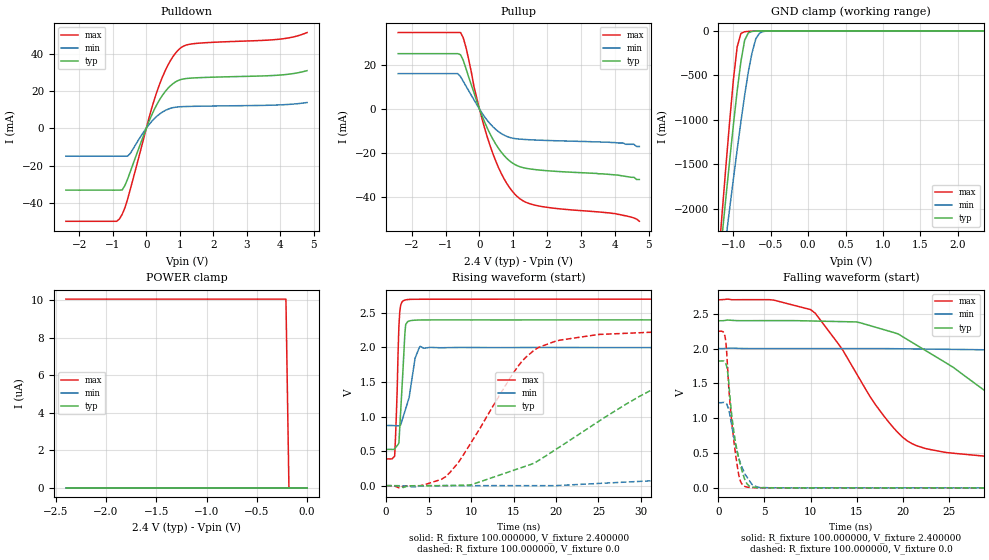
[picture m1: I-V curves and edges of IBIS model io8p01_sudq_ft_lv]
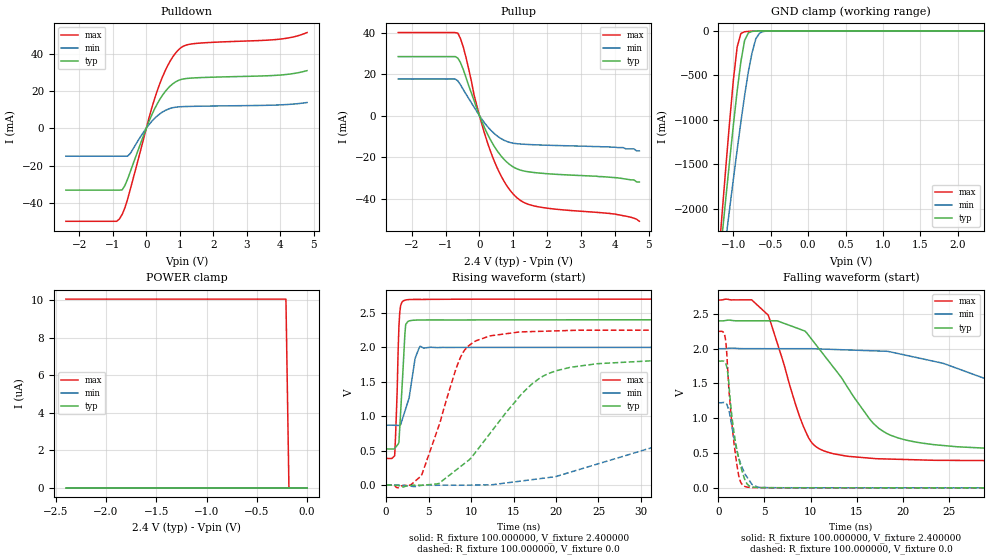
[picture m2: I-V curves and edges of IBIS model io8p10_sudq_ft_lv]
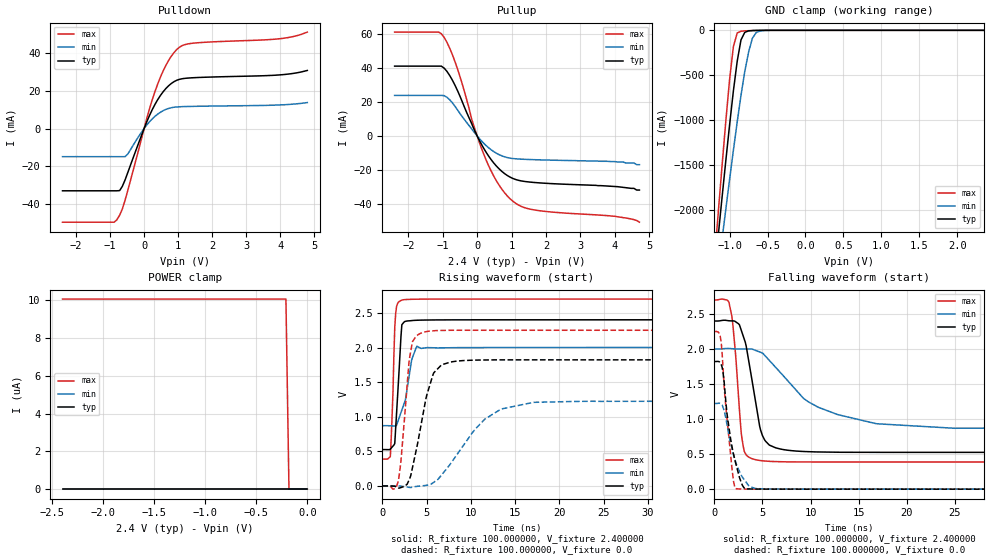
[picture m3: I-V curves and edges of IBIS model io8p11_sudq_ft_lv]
|   stm32f0_440_ufqfpn32 IBIS Model
[IBIS ver]   4.2
[File name]  stm32f0_440_ufqfpn32.ibs
[File Rev]   1.0
[Date]   15-5-2013
[Source] Data Created at STMicroelectronics
[Notes]   File originated from ELDO simulations.
[Disclaimer]  This information is for modeling purpose only and is
   not guaranted. The information is subject to change without
   notice.
[Copyright] Copyright 2015 STMicroelectronics Inc.
[Component] stm32f0_440_ufqfpn32
[Manufacturer] STMicroelectronics
[Package]
| variable   typ   min   max
R_pkg   0.0   NA   NA
L_pkg   0.0H   NA   NA
C_pkg   0.0F   NA   NA
[Pin] signal_name  model_name   R_pin   L_pin   C_pin
0   VSS_VSSA   GND   NA   NA   NA
1   VDD   POWER   0.03449   2.11E-09   6E-14
2   PF0   io8p_sudq_ft   0.029020556   1.54333E-09   3.22222E-14
3   PF1   io8p_sudq_ft   0.025738889   1.20333E-09   1.55556E-14
4   NRST  ioreset_tc_v33   0.024645   1.09E-09   1E-14
5   VDDA  POWER   0.024645   1.09E-09   1E-14
6   PA0   io8p_sudq_ft   0.025738889   1.20333E-09   1.55556E-14
7   PA1   io8p_sudq_ft   0.029020556   1.54333E-09   3.22222E-14
8   PA2   io8p_sudq_ft   0.03449   2.11E-09   6E-14
9   PA3   io8p_sudq_ft   0.03449   2.11E-09   6E-14
10   PA4   io8p_sudq_ft   0.029020556   1.54333E-09   3.22222E-14
11   PA5   io8p_sudq_ft   0.025738889   1.20333E-09   1.55556E-14
12   PA6   io8p_sudq_ft   0.024645   1.09E-09   1E-14
13   PA7   io8p_sudq_ft   0.024645   1.09E-09   1E-14
14   PB0   io8p_sudq_ft   0.025738889   1.20333E-09   1.55556E-14
15   PB1   io8p_sudq_ft   0.029020556   1.54333E-09   3.22222E-14
16   PB2   io8p_sudq_ft   0.03449   2.11E-09   6E-14
17   VDD   POWER   0.03449   2.11E-09   6E-14
18   PA8   io8p_sudq_ft   0.029020556   1.54333E-09   3.22222E-14
19   PA9   io8p_sudq_ft   0.025738889   1.20333E-09   1.55556E-14
20   PA10  io8p_sudq_ft   0.024645   1.09E-09   1E-14
21   PA11  io8p_sudq_ft   0.024645   1.09E-09   1E-14
22   PA12  io8p_sudq_ft   0.025738889   1.20333E-09   1.55556E-14
23   PA13  io8p_sudq_ft   0.029020556   1.54333E-09   3.22222E-14
24   PA14  io8p_sudq_ft   0.03449   2.11E-09   6E-14
25   PA15  io8p_sudq_ft   0.03449   2.11E-09   6E-14
26   PB3   io8p_sudq_ft   0.029020556   1.54333E-09   3.22222E-14
27   PB4   io8p_sudq_ft   0.025738889   1.20333E-09   1.55556E-14
28   PB5   io8p_sudq_ft   0.024645   1.09E-09   1E-14
29   PB6   io8p_sudq_i2cin_lv_ft   0.024645   1.09E-09   1E-14
30   PB7   io8p_sudq_i2cin_lv_ft   0.025738889   1.20333E-09   1.55556E-14
31   BOOT0 vpp_test_hv   0.029020556   1.54333E-09   3.22222E-14
32   PB8   io8p_sudq_i2cin_lv_ft   0.03449   2.11E-09   6E-14
[Model Selector] io8p_sudq_ft
io8p01_sudq_ft_pd_lv  "SPEED01 2P0V, PD=40kOhm"
io8p01_sudq_ft_pu_lv  "SPEED01 2P0V, PU=40kOhm"
io8p01_sudq_ft_lv  "SPEED01 2P0V"
io8p10_sudq_ft_pd_lv  "SPEED10 2P0V, PD=40kOhm"
io8p10_sudq_ft_pu_lv  "SPEED10 2P0V, PU=40kOhm"
io8p10_sudq_ft_lv  "SPEED10 2P0V"
io8p11_sudq_ft_pd_lv  "SPEED11 2P0V, PD=40kOhm"
io8p11_sudq_ft_pu_lv  "SPEED11 2P0V, PU=40kOhm"
io8p11_sudq_ft_lv  "SPEED11 2P0V"
io8p01_sudq_ft_pd  "SPEED01, PD=40kOhm"
io8p01_sudq_ft_pu  "SPEED01, PU=40kOhm"
io8p01_sudq_ft  "SPEED01"
io8p10_sudq_ft_pd  "SPEED10, PD=40kOhm"
io8p10_sudq_ft_pu  "SPEED10, PU=40kOhm"
io8p10_sudq_ft  "SPEED10"
io8p11_sudq_ft_pd  "SPEED11, PD=40kOhm"
io8p11_sudq_ft_pu  "SPEED11, PU=40kOhm"
io8p11_sudq_ft  "SPEED11"
[Model Selector] io8p_sudq_i2cin_lv_ft
io8p01_sudq_i2cin_lv_ft_pd_lv  "SPEED01 2P0V, PD=40kOhm"
io8p01_sudq_i2cin_lv_ft_pu_lv  "SPEED01 2P0V, PU=40kOhm"
io8p01_sudq_i2cin_lv_ft_lv  "SPEED01 2P0V"
io8p10_sudq_i2cin_lv_ft_pd_lv  "SPEED10 2P0V, PD=40kOhm"
io8p10_sudq_i2cin_lv_ft_pu_lv  "SPEED10 2P0V, PU=40kOhm"
io8p10_sudq_i2cin_lv_ft_lv  "SPEED10 2P0V"
io8p11_sudq_i2cin_lv_ft_pd_lv  "SPEED11 2P0V, PD=40kOhm"
io8p11_sudq_i2cin_lv_ft_pu_lv  "SPEED11 2P0V, PU=40kOhm"
io8p11_sudq_i2cin_lv_ft_lv  "SPEED11 2P0V"
io8p01_sudq_i2cin_lv_ft_pd  "SPEED01, PD=40kOhm"
io8p01_sudq_i2cin_lv_ft_pu  "SPEED01, PU=40kOhm"
io8p01_sudq_i2cin_lv_ft  "SPEED01"
io8p10_sudq_i2cin_lv_ft_pd  "SPEED10, PD=40kOhm"
io8p10_sudq_i2cin_lv_ft_pu  "SPEED10, PU=40kOhm"
io8p10_sudq_i2cin_lv_ft  "SPEED10"
io8p11_sudq_i2cin_lv_ft_pd  "SPEED11, PD=40kOhm"
io8p11_sudq_i2cin_lv_ft_pu  "SPEED11, PU=40kOhm"
io8p11_sudq_i2cin_lv_ft  "SPEED11"
[Model Selector] ioreset_tc_v33
ioreset_tc_v33_pu_lv  "IORESET 2V + PU=40kOhm"
ioreset_tc_v33_nopu_lv  "IORESET 2V"
ioreset_tc_v33_pu  "IORESET + PU=40kOhm"
ioreset_tc_v33_nopu  "IORESET"
[Model Selector] vpp_test_hv
vpp_test_hv_3p3  "Input Buffer"
vpp_test_hv_2p4  "Input Buffer 2P0V"
| Models and submodels in the file (42): io8p01_sudq_ft_pd_lv (I/O), io8p01_sudq_ft_pu_lv (I/O), io8p01_sudq_ft_lv (I/O), io8p10_sudq_ft_pd_lv (I/O), io8p10_sudq_ft_pu_lv (I/O), io8p10_sudq_ft_lv (I/O), io8p11_sudq_ft_pd_lv (I/O), io8p11_sudq_ft_pu_lv (I/O), io8p11_sudq_ft_lv (I/O), io8p01_sudq_ft_pd (I/O), io8p01_sudq_ft_pu (I/O), io8p01_sudq_ft (I/O), io8p10_sudq_ft_pd (I/O), io8p10_sudq_ft_pu (I/O), io8p10_sudq_ft (I/O), io8p11_sudq_ft_pd (I/O), io8p11_sudq_ft_pu (I/O), io8p11_sudq_ft (I/O), io8p01_sudq_i2cin_lv_ft_pd_lv (I/O), io8p01_sudq_i2cin_lv_ft_pu_lv (I/O), io8p01_sudq_i2cin_lv_ft_lv (I/O), io8p10_sudq_i2cin_lv_ft_pd_lv (I/O), io8p10_sudq_i2cin_lv_ft_pu_lv (I/O), io8p10_sudq_i2cin_lv_ft_lv (I/O), io8p11_sudq_i2cin_lv_ft_pd_lv (I/O), io8p11_sudq_i2cin_lv_ft_pu_lv (I/O), io8p11_sudq_i2cin_lv_ft_lv (I/O), io8p01_sudq_i2cin_lv_ft_pd (I/O), io8p01_sudq_i2cin_lv_ft_pu (I/O), io8p01_sudq_i2cin_lv_ft (I/O), io8p10_sudq_i2cin_lv_ft_pd (I/O), io8p10_sudq_i2cin_lv_ft_pu (I/O), io8p10_sudq_i2cin_lv_ft (I/O), io8p11_sudq_i2cin_lv_ft_pd (I/O), io8p11_sudq_i2cin_lv_ft_pu (I/O), io8p11_sudq_i2cin_lv_ft (I/O), ioreset_tc_v33_pu_lv (I/O_open_drain), ioreset_tc_v33_nopu_lv (I/O_open_drain), ioreset_tc_v33_pu (I/O_open_drain), ioreset_tc_v33_nopu (I/O_open_drain), vpp_test_hv_2p4 (Input), vpp_test_hv_3p3 (Input)
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|   Model io8p01_sudq_ft_lv
[Model]  io8p01_sudq_ft_lv
Model_type I/O
Polarity   Non-Inverting
Enable   Active-Low
Vinl =   0.720000V
Vinh =   1.680000V
Vmeas =  1.200000V
Cref =   50.000000pF
Rref =   100.000000M
Vref =   0.0V
C_comp   1.970100pF   1.887900pF   2.069400pF
[Temperature Range]   25.000000   0.125000k   -40.000000
[Pullup Reference]   2.400000V   2.000000V   2.700000V
[Pulldown Reference]   0.0V   0.0V   0.0V
[POWER Clamp Reference]   2.400000V   2.000000V   2.700000V
[GND Clamp Reference]   0.0V   0.0V   0.0V
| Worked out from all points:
|   slope of the pulldown table from 0 to 0.36 V, typ, clamps not added: 25.5 ohm
|   slope of the pullup table from 0 to 0.36 V, typ, clamps not added: 28.4 ohm
|   GND clamp passes 1 mA (typ) near -0.64 V on its own axis
|   rising waveform, R_fixture 100.000000, V_fixture 2.400000: 20-80 % time 499ps typ, 1.06ns min, 336ps max; typ from 0.525 V to 2.4 V
|   rising waveform, R_fixture 100.000000, V_fixture 0.0: 20-80 % time 14.5ns typ, 43.7ns min, 6.87ns max; typ from 0 V to 1.82 V
|   falling waveform, R_fixture 100.000000, V_fixture 2.400000: 20-80 % time 13ns typ, 32.3ns min, 7.05ns max; typ from 2.4 V to 0.525 V
|   falling waveform, R_fixture 100.000000, V_fixture 0.0: 20-80 % time 1.16ns typ, 1.39ns min, 931ps max; typ from 1.82 V to 0 V
[Pulldown]
|Voltage   I(typ)   I(min)   I(max)
-2.4V     -33.16mA   -14.98mA   -49.86mA
-880mV    -33.16mA   -14.98mA   -49.86mA
-800mV    -33.16mA   -14.98mA   -48.55mA
-640mV    -30.75mA   -14.98mA   -42.76mA
-480mV    -23.43mA   -13.57mA   -32.92mA
80mV      3.651mA    1.905mA    5.506mA
400mV     15.37mA    7.665mA    23.73mA
720mV     22.75mA    10.69mA    36.23mA
1.04V     26.18mA    11.57mA    43.27mA
1.52V     27.09mA    11.81mA    45.55mA
4V        28.55mA    12.55mA    47.81mA
4.8V      30.9mA     13.81mA    51.31mA
[Pullup]
|Voltage   I(typ)   I(min)   I(max)
-2.4V     25.21mA    16.13mA    34.79mA
-640mV    25.21mA    16.13mA    34.79mA
-560mV    24.72mA    14.75mA    34.79mA
-400mV    18.51mA    10.48mA    28.09mA
-160mV    7.322mA    4.15mA     10.02mA
80mV      -3.229mA   -1.94mA    -4.736mA
400mV     -13.82mA   -8.081mA   -20.45mA
800mV     -22.31mA   -12.38mA   -33.66mA
1.2V      -26.24mA   -13.65mA   -40.83mA
1.76V     -27.69mA   -14.12mA   -44.07mA
4V        -29.9mA    -15.2mA    -47.5mA
4.72V     -32mA      -17mA      -51mA
[GND_clamp]
|Voltage   I(typ)   I(min)   I(max)
-2.4V     -9.788A    -9.782A    -9.734A
-1.2V     -2.718A    -3.02A     -2.568A
-1.15V    -2.29A     -2.675A    -2.036A
-1.1V     -1.868A    -2.333A    -1.515A
-1.05V    -1.454A    -1.995A    -1.012A
-950mV    -674.5mA   -1.337A    -180.5mA
-900mV    -345.2mA   -1.023A    -29.72mA
-850mV    -106.4mA   -726mA     -10.13mA
-750mV    -6.396mA   -244mA     -4.026mA
-700mV    -2.558mA   -88.61mA   -2.329mA
-600mV    -416uA     -7.739mA   -368uA
2.35V     0A         0A         0A
[POWER_clamp]
|Voltage   I(typ)   I(min)   I(max)
-2.4V     0A         0A         10.06uA
-210mV    0A         0A         10.06uA
-180mV    0A         0A         0A
0V        0A         0A         0A
[Ramp]
| variable   typ   min   max
dV/dt_r  1.09308/14.53591n   0.73368/43.60005n   1.34946/6.86189n
dV/dt_f  1.12469/12.94342n   0.67781/32.23620n   1.38756/7.04174n
R_load = 100.000000
[Rising Waveform]
R_fixture= 100.000000
V_fixture= 2.400000
V_fixture_min= 2.000000
V_fixture_max= 2.700000
|time   V(typ)   V(min)   V(max)
0s        525.2mV    870.3mV    387.4mV
1.001ns   533.4mV    868.6mV    427.9mV
1.301ns   580.2mV    867mV      1.396V
1.502ns   618.9mV    866.4mV    2.308V
1.702ns   1.058V     877.1mV    2.607V
2.202ns   2.2V       1.075V     2.686V
2.703ns   2.383V     1.274V     2.696V
3.403ns   2.395V     1.844V     2.698V
4.004ns   2.398V     2.016V     2.698V
49.85ns   2.4V       2V         2.7V
[Rising Waveform]
R_fixture= 100.000000
V_fixture= 0.0
V_fixture_min= 0.0
V_fixture_max= 0.0
|time   V(typ)   V(min)   V(max)
0s        1.81nV     16.19nV    1.388nV
7.007ns   1.867mV    817.4uV    130.2mV
16.52ns   286.2mV    456uV      1.866V
20.02ns   528mV      1.164mV    2.095V
25.03ns   931.2mV    32.13mV    2.189V
37.04ns   1.629V     132.6mV    2.24V
54.55ns   1.791V     444.2mV    2.251V
84.08ns   1.821V     947.3mV    2.249V
106.1ns   1.822V     1.128V     2.249V
249.2ns   1.822V     1.223V     2.249V
[Falling Waveform]
R_fixture= 100.000000
V_fixture= 2.400000
V_fixture_min= 2.000000
V_fixture_max= 2.700000
|time   V(typ)   V(min)   V(max)
0s        2.4V       2V         2.7V
10.01ns   2.397V     2V         2.56V
15.02ns   2.383V     2V         1.637V
20.02ns   2.171V     1.997V     726.6mV
29.03ns   1.387V     1.983V     453.9mV
37.04ns   789.8mV    1.94V      415.8mV
52.55ns   592.4mV    1.669V     394.5mV
72.57ns   546.2mV    1.209V     388.6mV
99.1ns    528mV      969.1mV    387.4mV
249.2ns   525.2mV    870.3mV    387.4mV
[Falling Waveform]
R_fixture= 100.000000
V_fixture= 0.0
V_fixture_min= 0.0
V_fixture_max= 0.0
|time   V(typ)   V(min)   V(max)
0s        1.822V     1.223V     2.249V
700.7ps   1.802V     1.223V     2.18V
800.8ps   1.785V     1.216V     2.097V
1.001ns   1.655V     1.166V     1.704V
1.201ns   1.378V     1.071V     1.289V
1.902ns   616.6mV    591.6mV    436.6mV
2.302ns   369.3mV    388.2mV    131.7mV
2.903ns   108.1mV    191.2mV    18.1mV
4.705ns   2.197mV    4.103mV    1.139mV
49.85ns   1.81nV     16.19nV    1.388nV
|   Model io8p10_sudq_ft_lv
[Model]  io8p10_sudq_ft_lv
Model_type I/O
Polarity   Non-Inverting
Enable   Active-Low
Vinl =   0.720000V
Vinh =   1.680000V
Vmeas =  1.200000V
Cref =   50.000000pF
Rref =   100.000000M
Vref =   0.0V
C_comp   1.970100pF   1.887900pF   2.069400pF
[Temperature Range]   25.000000   0.125000k   -40.000000
[Pullup Reference]   2.400000V   2.000000V   2.700000V
[Pulldown Reference]   0.0V   0.0V   0.0V
[POWER Clamp Reference]   2.400000V   2.000000V   2.700000V
[GND Clamp Reference]   0.0V   0.0V   0.0V
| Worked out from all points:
|   slope of the pulldown table from 0 to 0.36 V, typ, clamps not added: 25.5 ohm
|   slope of the pullup table from 0 to 0.36 V, typ, clamps not added: 28.4 ohm
|   GND clamp passes 1 mA (typ) near -0.64 V on its own axis
|   rising waveform, R_fixture 100.000000, V_fixture 2.400000: 20-80 % time 501ps typ, 1.06ns min, 336ps max; typ from 0.525 V to 2.4 V
|   rising waveform, R_fixture 100.000000, V_fixture 0.0: 20-80 % time 7.32ns typ, 21.7ns min, 3.52ns max; typ from 0 V to 1.82 V
|   falling waveform, R_fixture 100.000000, V_fixture 2.400000: 20-80 % time 6.27ns typ, 18.5ns min, 3.33ns max; typ from 2.4 V to 0.525 V
|   falling waveform, R_fixture 100.000000, V_fixture 0.0: 20-80 % time 1.16ns typ, 1.4ns min, 914ps max; typ from 1.82 V to 0 V
[Pulldown]
|Voltage   I(typ)   I(min)   I(max)
-2.4V     -33.16mA   -14.98mA   -49.86mA
-880mV    -33.16mA   -14.98mA   -49.86mA
-800mV    -33.16mA   -14.98mA   -48.55mA
-640mV    -30.75mA   -14.98mA   -42.76mA
-480mV    -23.43mA   -13.57mA   -32.92mA
80mV      3.651mA    1.905mA    5.506mA
400mV     15.37mA    7.665mA    23.73mA
720mV     22.75mA    10.69mA    36.23mA
1.04V     26.18mA    11.57mA    43.27mA
1.52V     27.09mA    11.81mA    45.55mA
4V        28.55mA    12.55mA    47.81mA
4.8V      30.9mA     13.81mA    51.31mA
[Pullup]
|Voltage   I(typ)   I(min)   I(max)
-2.4V     28.57mA    17.75mA    40.17mA
-720mV    28.57mA    17.75mA    40.17mA
-640mV    27.85mA    16.83mA    39.88mA
-480mV    22.38mA    12.65mA    33.22mA
-80mV     3.427mA    2.066mA    4.957mA
160mV     -6.219mA   -3.715mA   -9.137mA
320mV     -11.51mA   -6.781mA   -16.98mA
720mV     -21mA      -11.8mA    -31.54mA
1.12V     -25.77mA   -13.54mA   -39.82mA
1.76V     -27.69mA   -14.12mA   -44.07mA
4V        -29.9mA    -15.2mA    -47.5mA
4.72V     -32mA      -17mA      -51mA
[GND_clamp]
|Voltage   I(typ)   I(min)   I(max)
-2.4V     -9.788A    -9.782A    -9.734A
-1.2V     -2.718A    -3.02A     -2.568A
-1.15V    -2.29A     -2.675A    -2.036A
-1.1V     -1.868A    -2.333A    -1.515A
-1.05V    -1.454A    -1.995A    -1.012A
-950mV    -674.5mA   -1.337A    -180.5mA
-900mV    -345.2mA   -1.023A    -29.72mA
-850mV    -106.4mA   -726mA     -10.13mA
-750mV    -6.396mA   -244mA     -4.026mA
-700mV    -2.558mA   -88.61mA   -2.329mA
-600mV    -416uA     -7.739mA   -368uA
2.35V     0A         0A         0A
[POWER_clamp]
|Voltage   I(typ)   I(min)   I(max)
-2.4V     0A         0A         10.06uA
-210mV    0A         0A         10.06uA
-180mV    0A         0A         0A
0V        0A         0A         0A
[Ramp]
| variable   typ   min   max
dV/dt_r  1.09308/7.31082n   0.73308/21.71145n   1.34964/3.51759n
dV/dt_f  1.12481/6.26349n   0.67631/18.49686n   1.38754/3.32485n
R_load = 100.000000
[Rising Waveform]
R_fixture= 100.000000
V_fixture= 2.400000
V_fixture_min= 2.000000
V_fixture_max= 2.700000
|time   V(typ)   V(min)   V(max)
0s        525.2mV    870.3mV    387.4mV
1.001ns   533.2mV    868.7mV    426.9mV
1.301ns   579.1mV    867.1mV    1.388V
1.502ns   617.1mV    866.5mV    2.304V
1.702ns   1.054V     877mV      2.604V
2.202ns   2.189V     1.072V     2.684V
2.603ns   2.379V     1.227V     2.693V
3.403ns   2.395V     1.838V     2.696V
4.004ns   2.397V     2.017V     2.696V
49.85ns   2.4V       2V         2.7V
[Rising Waveform]
R_fixture= 100.000000
V_fixture= 0.0
V_fixture_min= 0.0
V_fixture_max= 0.0
|time   V(typ)   V(min)   V(max)
0s        1.81nV     16.19nV    1.388nV
2.803ns   -3.281mV   -14.07mV   -1.578mV
4.204ns   -1.834mV   -2.504mV   153.3mV
8.809ns   274.6mV    -1.375mV   1.87V
12.21ns   748.9mV    4.656mV    2.166V
18.02ns   1.547V     92.84mV    2.232V
24.82ns   1.763V     304.5mV    2.249V
40.24ns   1.817V     861.6mV    2.249V
51.85ns   1.822V     1.107V     2.249V
99.7ns    1.822V     1.223V     2.249V
[Falling Waveform]
R_fixture= 100.000000
V_fixture= 2.400000
V_fixture_min= 2.000000
V_fixture_max= 2.700000
|time   V(typ)   V(min)   V(max)
0s        2.4V       2V         2.7V
3.604ns   2.401V     2V         2.703V
5.405ns   2.402V     2V         2.482V
9.81ns    2.189V     2V         715.2mV
14.01ns   1.448V     1.982V     453.6mV
18.22ns   786.7mV    1.963V     414.6mV
25.83ns   591.3mV    1.722V     393.9mV
36.04ns   545.2mV    1.277V     387.5mV
53.05ns   528.1mV    942.3mV    387.4mV
99.7ns    525.2mV    870.3mV    387.4mV
[Falling Waveform]
R_fixture= 100.000000
V_fixture= 0.0
V_fixture_min= 0.0
V_fixture_max= 0.0
|time   V(typ)   V(min)   V(max)
0s        1.822V     1.223V     2.249V
700.7ps   1.802V     1.222V     2.18V
800.8ps   1.785V     1.215V     2.098V
1.001ns   1.656V     1.165V     1.707V
1.401ns   1.093V     924.2mV    997.1mV
1.902ns   616.8mV    592mV      421.8mV
2.302ns   368.5mV    388.7mV    122.4mV
2.903ns   107.4mV    191.2mV    17.72mV
4.705ns   2.748mV    4.47mV     1.93mV
49.85ns   1.81nV     16.19nV    1.388nV
|   Model io8p11_sudq_ft_lv
[Model]  io8p11_sudq_ft_lv
Model_type I/O
Polarity   Non-Inverting
Enable   Active-Low
Vinl =   0.720000V
Vinh =   1.680000V
Vmeas =  1.200000V
Cref =   50.000000pF
Rref =   100.000000M
Vref =   0.0V
C_comp   1.970100pF   1.887900pF   2.069400pF
[Temperature Range]   25.000000   0.125000k   -40.000000
[Pullup Reference]   2.400000V   2.000000V   2.700000V
[Pulldown Reference]   0.0V   0.0V   0.0V
[POWER Clamp Reference]   2.400000V   2.000000V   2.700000V
[GND Clamp Reference]   0.0V   0.0V   0.0V
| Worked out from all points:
|   slope of the pulldown table from 0 to 0.36 V, typ, clamps not added: 25.5 ohm
|   slope of the pullup table from 0 to 0.36 V, typ, clamps not added: 28.4 ohm
|   GND clamp passes 1 mA (typ) near -0.64 V on its own axis
|   rising waveform, R_fixture 100.000000, V_fixture 2.400000: 20-80 % time 509ps typ, 1.05ns min, 338ps max; typ from 0.525 V to 2.4 V
|   rising waveform, R_fixture 100.000000, V_fixture 0.0: 20-80 % time 1.79ns typ, 4.5ns min, 865ps max; typ from 0 V to 1.82 V
|   falling waveform, R_fixture 100.000000, V_fixture 2.400000: 20-80 % time 1.38ns typ, 6.07ns min, 772ps max; typ from 2.4 V to 0.525 V
|   falling waveform, R_fixture 100.000000, V_fixture 0.0: 20-80 % time 1.17ns typ, 1.4ns min, 851ps max; typ from 1.82 V to 0 V
[Pulldown]
|Voltage   I(typ)   I(min)   I(max)
-2.4V     -33.16mA   -14.98mA   -49.86mA
-880mV    -33.16mA   -14.98mA   -49.86mA
-800mV    -33.16mA   -14.98mA   -48.55mA
-640mV    -30.75mA   -14.98mA   -42.76mA
-480mV    -23.43mA   -13.57mA   -32.92mA
80mV      3.651mA    1.905mA    5.506mA
400mV     15.37mA    7.665mA    23.73mA
720mV     22.75mA    10.69mA    36.23mA
1.04V     26.18mA    11.57mA    43.27mA
1.52V     27.09mA    11.81mA    45.55mA
4V        28.55mA    12.55mA    47.81mA
4.8V      30.9mA     13.81mA    51.31mA
[Pullup]
|Voltage   I(typ)   I(min)   I(max)
-2.4V     41.23mA    23.94mA    61.35mA
-1.12V    41.23mA    23.94mA    61.35mA
-960mV    40.07mA    23.8mA     58.26mA
-800mV    35.78mA    21.41mA    51.94mA
-560mV    26.31mA    15mA       38.91mA
-160mV    7.322mA    4.15mA     10.02mA
240mV     -8.977mA   -5.327mA   -13.21mA
640mV     -19.5mA    -11.09mA   -29.16mA
1.04V     -25.16mA   -13.38mA   -38.61mA
1.68V     -27.56mA   -14.07mA   -43.82mA
4V        -29.9mA    -15.2mA    -47.5mA
4.72V     -32mA      -17mA      -51mA
[GND_clamp]
|Voltage   I(typ)   I(min)   I(max)
-2.4V     -9.788A    -9.782A    -9.734A
-1.2V     -2.718A    -3.02A     -2.568A
-1.15V    -2.29A     -2.675A    -2.036A
-1.1V     -1.868A    -2.333A    -1.515A
-1.05V    -1.454A    -1.995A    -1.012A
-950mV    -674.5mA   -1.337A    -180.5mA
-900mV    -345.2mA   -1.023A    -29.72mA
-850mV    -106.4mA   -726mA     -10.13mA
-750mV    -6.396mA   -244mA     -4.026mA
-700mV    -2.558mA   -88.61mA   -2.329mA
-600mV    -416uA     -7.739mA   -368uA
2.35V     0A         0A         0A
[POWER_clamp]
|Voltage   I(typ)   I(min)   I(max)
-2.4V     0A         0A         10.06uA
-210mV    0A         0A         10.06uA
-180mV    0A         0A         0A
0V        0A         0A         0A
[Ramp]
| variable   typ   min   max
dV/dt_r  1.09302/1.79298n   0.73362/4.49721n   1.34964/0.86038n
dV/dt_f  1.12491/1.37677n   0.67799/6.06609n   1.38752/0.77139n
R_load = 100.000000
[Rising Waveform]
R_fixture= 100.000000
V_fixture= 2.400000
V_fixture_min= 2.000000
V_fixture_max= 2.700000
|time   V(typ)   V(min)   V(max)
0s        525.2mV    870.3mV    387.4mV
900.9ps   532.8mV    868.8mV    423.8mV
1.201ns   575.8mV    867.5mV    1.36V
1.401ns   611.9mV    867.1mV    2.288V
1.602ns   1.043V     877.1mV    2.592V
2.202ns   2.329V     1.096V     2.685V
2.603ns   2.378V     1.242V     2.693V
3.303ns   2.389V     1.815V     2.697V
3.904ns   2.394V     2.018V     2.698V
49.85ns   2.4V       2V         2.7V
[Rising Waveform]
R_fixture= 100.000000
V_fixture= 0.0
V_fixture_min= 0.0
V_fixture_max= 0.0
|time   V(typ)   V(min)   V(max)
0s        -34.42uV   -16.09uV   -30.78uV
1.802ns   -29.45mV   -740.6uV   67.32mV
3.103ns   111mV      -21.81mV   1.872V
3.403ns   265.9mV    -17.89mV   2.083V
4.505ns   973.7mV    1.595mV    2.215V
5.706ns   1.601V     43.39mV    2.241V
6.707ns   1.75V      161.3mV    2.247V
10.71ns   1.818V     849.4mV    2.249V
13.61ns   1.822V     1.116V     2.249V
49.85ns   1.822V     1.223V     2.249V
[Falling Waveform]
R_fixture= 100.000000
V_fixture= 2.400000
V_fixture_min= 2.000000
V_fixture_max= 2.700000
|time   V(typ)   V(min)   V(max)
0s        2.4V       2V         2.7V
1.502ns   2.403V     2.008V     2.671V
1.902ns   2.401V     2.004V     2.368V
2.903ns   2.223V     2.001V     690.6mV
4.004ns   1.477V     1.995V     431mV
5.205ns   706.9mV    1.914V     401.7mV
7.508ns   557.6mV    1.566V     389.5mV
10.81ns   530.8mV    1.169V     387.3mV
16.82ns   525.4mV    935mV      387.5mV
49.85ns   525.2mV    870.3mV    387.4mV
[Falling Waveform]
R_fixture= 100.000000
V_fixture= 0.0
V_fixture_min= 0.0
V_fixture_max= 0.0
|time   V(typ)   V(min)   V(max)
0s        1.822V     1.223V     2.249V
700.7ps   1.784V     1.214V     2.101V
1.101ns   1.383V     1.071V     1.306V
1.301ns   1.083V     925.1mV    1.011V
1.802ns   626.2mV    594.7mV    324.2mV
2.102ns   432.6mV    434mV      34.1mV
2.302ns   323.4mV    348.4mV    4.72mV
3.103ns   15.77mV    135.4mV    1.387mV
4.605ns   1.159mV    5.956mV    462.6uV
49.85ns   -34.42uV   -16.09uV   -30.78uV
